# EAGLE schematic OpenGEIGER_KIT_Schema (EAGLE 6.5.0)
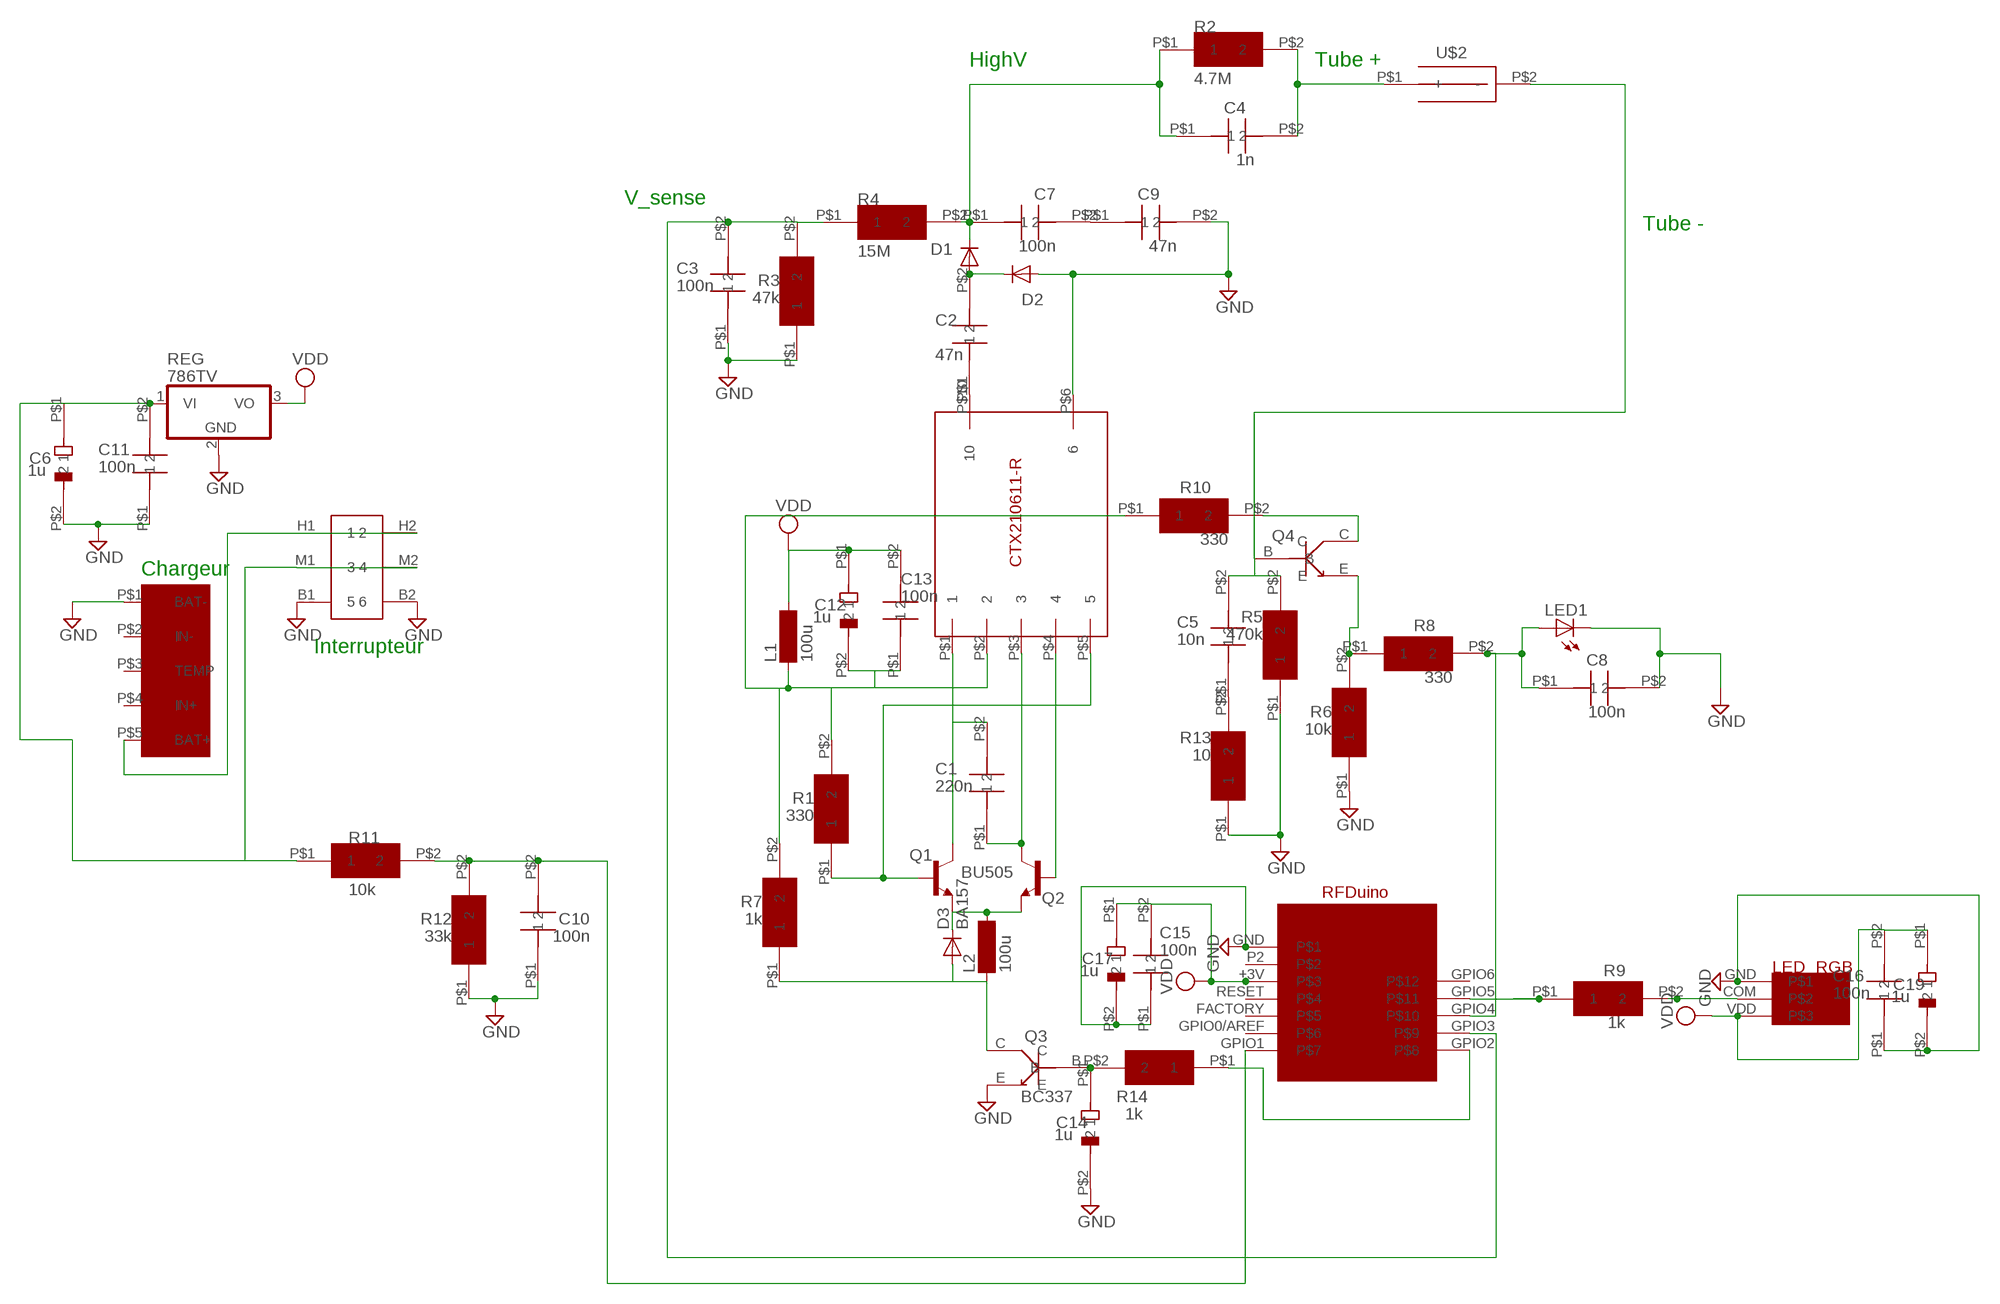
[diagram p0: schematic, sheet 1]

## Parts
C1  220n  MY_CONDO  [MY_CONDO]
C2  47n  MY_CONDO  [MY_CONDO]
C3  100n  MY_CONDO  [MY_CONDO]
C4  1n  MY_CONDO  [MY_CONDO]
C5  10n  MY_CONDO  [MY_CONDO]
C6  1u  MY_CONDO_CH  [MY_CONDO_CH]
C7  100n  MY_CONDO  [MY_CONDO]
C8  100n  MY_CONDO  [MY_CONDO]
C9  47n  MY_CONDO  [MY_CONDO]
C10  100n  MY_CONDO  [MY_CONDO]
C11  100n  MY_CONDO  [MY_CONDO]
C12  1u  MY_CONDO_CH  [MY_CONDO_CH]
C13  100n  MY_CONDO  [MY_CONDO]
C14  1u  MY_CONDO_CH  [MY_CONDO_CH]
C15  100n  MY_CONDO  [MY_CONDO]
C16  100n  MY_CONDO  [MY_CONDO]
C17  1u  MY_CONDO_CH  [MY_CONDO_CH]
C19  1u  MY_CONDO_CH  [MY_CONDO_CH]
D1  1N5060GP  [DO15-12]
D2  1N5060GP  [DO15-12]
D3  BA157  [P1-10]
L1  100u  SD8  [SD8]
L2  100u  SD8  [SD8]
LED1  LEDB155  [Q62902-B155]
Q1  BU505  2SC1306  [TO220BV]
Q2  BU505  2SC1306  [TO220BV]
Q3  BC337  MY_TO92  [MY_TO92]
Q4  BC337  MY_TO92  [MY_TO92]
R1  330  MY_RESISTANCE  [MY_RESISTANCE]
R2  4.7M  MY_BIG_R  [MY_BIG_R]
R3  47k  MY_RESISTANCE  [MY_RESISTANCE]
R4  15M  MY_BIG_R  [MY_BIG_R]
R5  470k  MY_RESISTANCE  [MY_RESISTANCE]
R6  10k  MY_RESISTANCE  [MY_RESISTANCE]
R7  1k  MY_RESISTANCE  [MY_RESISTANCE]
R8  330  MY_RESISTANCE  [MY_RESISTANCE]
R9  1k  MY_RESISTANCE  [MY_RESISTANCE]
R10  330  MY_RESISTANCE  [MY_RESISTANCE]
R11  10k  MY_RESISTANCE  [MY_RESISTANCE]
R12  33k  MY_RESISTANCE  [MY_RESISTANCE]
R13  10  MY_RESISTANCE  [MY_RESISTANCE]
R14  1k  MY_RESISTANCE  [MY_RESISTANCE]
REG  786TV  [TO220V]
U$1  CCFL_TRANSFO  [CCFL_TRANSFO]
U$2  TUBE  [TUBE]
U$3  ANTONYO  [ANTONYO]  (not placed on a sheet)
U$4  INTERRUPTEUR  [INTERRUPTEUR]
U$5  RFDUINO  [RFDUINO]
U$6  CHARGEUR  [CHARGEUR]
U$7  LED_RGB  [LED_RGB]

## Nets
CHARGEUR+: U$4.H1 U$4.H2 U$6.P$5(BAT+)
COUPS: C8.P$1 LED1.A R8.P$2 U$5.GPIO4
GND: C3.P$1 C6.P$2 C8.P$2 C9.P$2 C10.P$1 C11.P$1 C14.P$2 C15.P$1 C16.P$1 C17.P$2 C19.P$2 D2.A LED1.K(C) Q3.E R3.P$1 R5.P$1 R6.P$1 R12.P$1 R13.P$1 REG.2(GND) U$1.P$6 U$4.B1 U$4.B2 U$5.GND U$6.P$1(BAT-) U$7.GND
HIGH_V: C4.P$1 C7.P$1 D1.C R2.P$1 R4.P$2
N$1: R9.P$1 U$5.GPIO5
N$2: C7.P$2 C9.P$1
N$3: C2.P$2 D1.A D2.C
N$4: Q1.1(B) R1.P$1 U$1.P$5
N$5: D3.A L2.1 Q3.C R7.P$1
N$6: C5.P$2 Q4.B R5.P$2 U$2.P$2(-)
N$7: R9.P$2 U$7.COM
N$9: Q2.1(B) U$1.P$4
N$10: C10.P$2 R11.P$2 R12.P$2 U$5.GPIO1
N$11: C5.P$1 R13.P$2
N$12: C4.P$2 R2.P$2 U$2.P$1(+)
N$15: Q4.E R6.P$2 R8.P$1
N$17: C1.P$2 Q1.2(C) U$1.P$1
N$18: C14.P$1 Q3.B R14.P$2
N$19: Q4.C R10.P$2
N$22: D3.C L2.2 Q1.3(E) Q2.3(E)
N$23: C1.P$1 Q2.2(C) U$1.P$3
N$26: R14.P$1 U$5.GPIO2
N$28: C2.P$1 U$1.P$10
V_SENSE: C3.P$2 R3.P$2 R4.P$1 U$5.GPIO3
VDD_POST_BOBINE: C12.P$2 C13.P$1 L1.1 R1.P$2 R7.P$2 R10.P$1 U$1.P$2
VDD_PRE_REGULATOR: C6.P$1 C11.P$2 R11.P$1 REG.1(VI) U$4.M1 U$4.M2
VDD_PRé_BOBINE: C12.P$1 C13.P$2 C15.P$2 C16.P$2 C17.P$1 C19.P$1 L1.2 REG.3(VO) U$5.+3V U$7.VDD ; supply symbol labelled VDD
Unconnected: U$5.FACTORY U$5.GPIO0/AREF U$5.GPIO6 U$5.P2 U$5.RESET U$6.P$2(IN-) U$6.P$3(TEMP) U$6.P$4(IN+)

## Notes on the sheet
- HighV | Tube +
- V_sense
- Tube -
- Chargeur
- Interrupteur

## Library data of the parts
C1-C5 C7-C11 C13 C15 C16 = openGeiger:MY_CONDO
C6 C12 C14 C17 C19 = openGeiger:MY_CONDO_CH
D1 D2 = diode:1N5060GP: DIODE
D3 = diode:BA157: DIODE
L1 L2 = inductor-neosid:SD8: INDUCTOR; OC_FARNELL: unknown; OC_NEWARK: unknown
LED1 = led:LED: LED
Q1 Q2 = transistor:2SC1306: NPN Transistor Final RF Power Outupt Source: 2sc1306.pdf
Q3 Q4 = openGeiger:MY_TO92
R1 R3 R5-R14 = openGeiger:MY_RESISTANCE
R2 R4 = openGeiger:MY_BIG_R
REG = linear:78*: Positive VOLTAGE REGULATOR Source: http://cache.national.com/ds/LM/LM78L05.pdf http://www.fairchildsemi.com/ds/LM/LM7805.pdf
U$1 = openGeiger:CCFL_TRANSFO
U$2 = openGeiger:TUBE
U$3 = openGeiger:ANTONYO
U$4 = openGeiger:INTERRUPTEUR
U$5 = openGeiger:RFDUINO
U$6 = openGeiger:CHARGEUR
U$7 = openGeiger:LED_RGB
